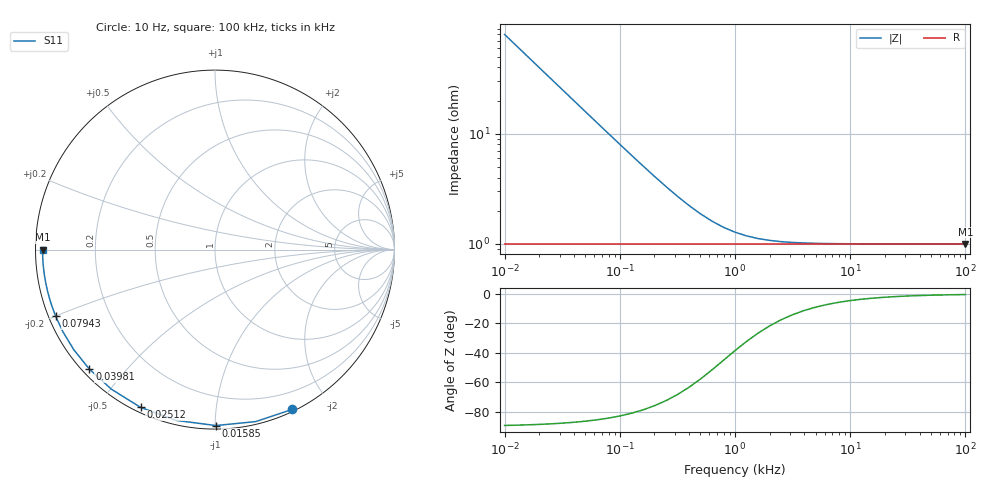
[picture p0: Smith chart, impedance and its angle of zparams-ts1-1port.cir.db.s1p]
# Hz Z DB R 50
!  Freq  magdbZ11  angZ11
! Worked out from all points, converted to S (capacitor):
!   41 points, 10 Hz to 100 kHz, reference 50 ohm
!   read as one part to ground: C = 200 uF near 10 Hz
!   lowest |Z| = 1 ohm at 100 kHz (marker M1)
!   S11 on the Smith chart (normalised r, x): 10 Hz: 0.02, -1.59; 15.85 Hz: 0.02, -1.00; 25.12 Hz: 0.02, -0.63; 39.81 Hz: 0.02, -0.40; 79.43 Hz: 0.02, -0.20; 100 kHz: 0.02, -0.00
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10  4.04 -89.3
12.58925  2.04 -89.1
15.84893  0.04 -88.9
19.95262  -1.96 -88.6
25.11886  -3.96 -88.2
31.62278  -5.96 -87.7
39.81072  -7.95 -87.1
50.11872  -9.95 -86.4
63.09573  -11.94 -85.5
79.43282  -13.92 -84.3
100  -15.90 -82.8
125.8925  -17.86 -81.0
158.4893  -19.79 -78.7
199.5262  -21.70 -75.9
251.1886  -23.55 -72.5
316.2278  -25.33 -68.3
398.1072  -26.99 -63.4
501.1872  -28.51 -57.8
630.9573  -29.85 -51.6
794.3282  -30.96 -45.1
1000  -31.85 -38.5
1258.925  -32.52 -32.3
1995.262  -33.34 -21.7
3981.072  -33.81 -11.3
6309.573  -33.91 -7.2
12589.25  -33.96 -3.6
39810.72  -33.98 -1.1
100000  -33.98 -0.5
